TYPE CKD_OUT :
STRUCT
	Control_Mode	:	USINT	;
	Process_Setpoint	:	REAL	;
	Position_Setpoint	:	REAL	;
	Exh_Rate	:	REAL	;
	Active_Controller	:	USINT	;
	Slow_exhaust_control_arrival_pressure	:	REAL	;

END_STRUCT
END_TYPE
